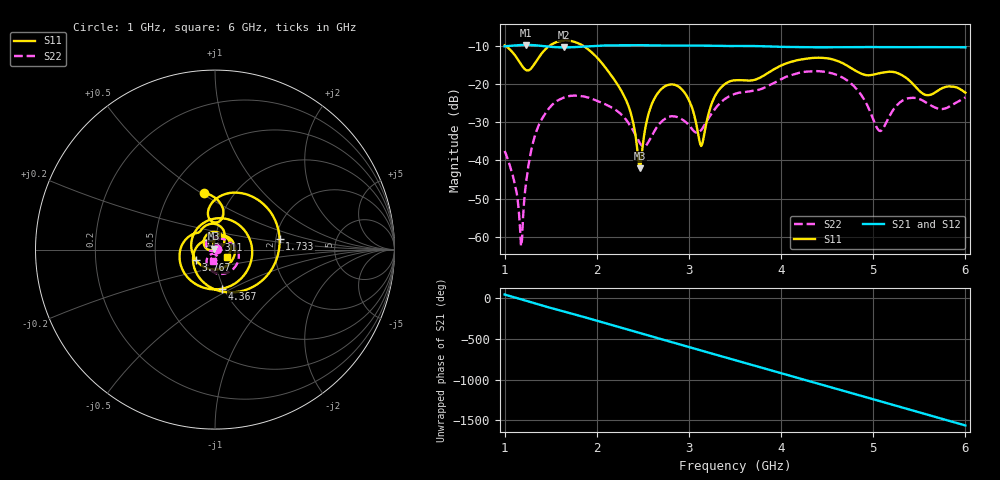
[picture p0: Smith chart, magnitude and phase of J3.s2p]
!Agilent Technologies,E8364B,MY43040528,A.07.50.67
!Agilent E8364B: A.07.50.67
!Date: Sunday, March 01, 2026 15:23:09
!Correction: S11(Full 2 Port(1,2))
!S21(Full 2 Port(1,2))
!S12(Full 2 Port(1,2))
!S22(Full 2 Port(1,2))
!S2P File: Measurements: S11, S21, S12, S22:
# Hz S  dB  R 50
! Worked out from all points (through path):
!   451 points, 1 GHz to 6 GHz, reference 50 ohm
!   highest |S21| = -9.71 dB at 1.233 GHz (marker M1); lowest = -10.4 dB at 1.644 GHz (marker M2)
!   group delay of S21, straight-line fit = 892 ps
!   lowest |S11| = -42.1 dB at 2.467 GHz (marker M3), VSWR 1.02, Z = 49.4 + j0.511 ohm
!   |S11| at or under -10 dB: 1.01 GHz to 1.484 GHz (474.6 MHz wide, 38.1 % of centre); 1.855 GHz to end of sweep
!   |S22| runs from -62.5 to -16.6 dB; largest |S21 - S12| = 0.0015
!   S11 on the Smith chart (normalised r, x): 1 GHz: 0.73, +0.51; 1.733 GHz: 2.10, +0.29; 2.311 GHz: 0.92, +0.10; 3.767 GHz: 0.80, -0.10; 4.367 GHz: 0.98, -0.45; 6 GHz: 1.13, -0.10
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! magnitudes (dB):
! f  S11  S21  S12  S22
! 1 GHz  -9.9  -10.1  -10.1  -37.5
! 1.111 GHz  -12.4  -9.9  -9.9  -46.3
! 1.178 GHz  -14.8  -9.7  -9.8  -62.5
! 1.233 GHz  -16.3  -9.7  -9.7  -45.6
! 1.378 GHz  -12.7  -9.9  -9.9  -30.4
! 1.644 GHz  -8.6  -10.4  -10.4  -23.5
! 1.733 GHz  -8.8  -10.3  -10.4  -23.0
! 1.844 GHz  -9.8  -10.2  -10.2  -23.2
! 2.311 GHz  -23.8  -9.8  -9.8  -29.1
! 2.467 GHz  -42.1  -9.8  -9.8  -35.4
! 2.667 GHz  -22.2  -9.9  -9.9  -30.8
! 2.933 GHz  -21.6  -9.9  -9.9  -29.4
! 3.133 GHz  -36.2  -9.9  -9.9  -32.0
! 3.289 GHz  -22.9  -10.0  -10.0  -26.3
! 3.5 GHz  -19.0  -10.0  -10.0  -22.5
! 3.767 GHz  -18.4  -10.0  -10.1  -21.4
! 4.344 GHz  -13.1  -10.3  -10.4  -16.6
! 4.367 GHz  -13.1  -10.3  -10.4  -16.6
! 4.767 GHz  -15.9  -10.3  -10.3  -20.0
! 5.067 GHz  -17.1  -10.3  -10.3  -32.2
! 5.167 GHz  -16.8  -10.3  -10.4  -28.8
! 6 GHz  -22.2  -10.3  -10.4  -23.5
